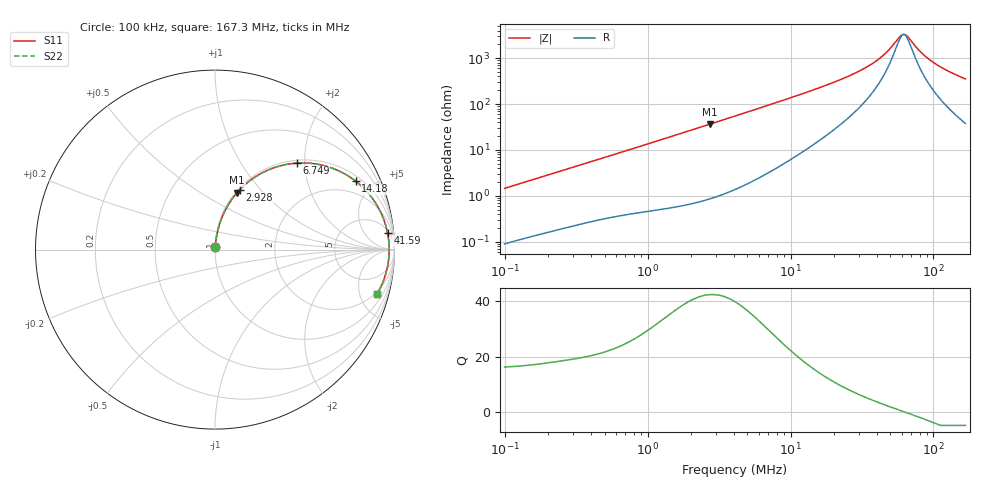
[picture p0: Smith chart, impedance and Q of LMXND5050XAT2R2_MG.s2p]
! LMXND5050XAT2R2_MG  S-PARAMETER MODEL  ( General Type )
! Model Generated by TAIYO YUDEN Corporation (https://www.yuden.co.jp/en/)
! Version 1.0
! TAIYO YUDEN Control No. 191023NI43SB-FBB
! Copyright(c) 2019 TAIYO YUDEN CO.,LTD. All Rights Reserved.
! Product Description (link to TY-COMPAS)
! https://ds.yuden.co.jp/TYCOMPAS/or/detail?pn=LMXND5050XAT2R2NMG&u=M
! Products Name : Inductors
! Characteristics :
!  Inductance : 2.2 uH , SRF(min) : 46 MHz , DC Resistance(max) : 0.0299 Ohm
!  Rated Current : Saturation :4200 mA , Temp Rise : 3500 mA (40 degC)
!  Case Size : 4.9 x 4.9 / 0.193 x 0.193 [mm/inch] , Thickness : 3.1 / 0.122 [mm/inch]
!  (Conditions: Temperature = 25 degC , DC Bias Current/Voltage = 0A / 0V)
! External Node Assignments :
!  1  o---GGG---o  2
! GND o---------o GND
! Frequency Range : 0.1MHz  -  167.251077MHz  [ 402 STEP ]
# MHz S RI R 50
! Freq[MHz].  S11 Real  S11 Imag  S21 Real  S21 Imag  S12 Real  S12 Imag  S22 Real  S22 Imag
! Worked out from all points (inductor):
!   401 points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, 100 kHz to 167.3 MHz, reference 50 ohm
!   read as one part in series: L = 2.29 uH near 103.8 kHz
!   highest Q = 42.5 at 2.719 MHz (marker M1), where L = 2.13 uH
!   self-resonance near 61.96 MHz
!   S11 on the Smith chart (normalised r, x): 100 kHz: 1.00, +0.03; 2.928 MHz: 1.02, +0.78; 6.749 MHz: 1.06, +1.82; 14.18 MHz: 1.25, +3.97; 41.59 MHz: 7, +18; 167.3 MHz: 1.75, -7.01
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0.1  0.00111 0.0145  0.9989 -0.0145  0.9989 -0.0145  0.00111 0.0145
0.346668  0.00474 0.0478  0.9953 -0.0478  0.9953 -0.0478  0.00474 0.0478
1.20179  0.03 0.1558  0.97 -0.1558  0.97 -0.1558  0.03 0.1558
2.718937  0.1225 0.3163  0.8775 -0.3163  0.8775 -0.3163  0.1225 0.3163
2.928417  0.1388 0.3342  0.8612 -0.3342  0.8612 -0.3342  0.1388 0.3342
4.166227  0.2431 0.4165  0.7569 -0.4165  0.7569 -0.4165  0.2431 0.4165
6.749349  0.4546 0.4818  0.5454 -0.4818  0.5454 -0.4818  0.4546 0.4818
9.602225  0.6267 0.4624  0.3733 -0.4624  0.3733 -0.4624  0.6267 0.4624
14.17747  0.7841 0.3811  0.2159 -0.3811  0.2159 -0.3811  0.7841 0.3811
19.43533  0.8707 0.2939  0.1293 -0.2939  0.1293 -0.2939  0.8707 0.2939
27.14211  0.9267 0.2008  0.0733 -0.2008  0.0733 -0.2008  0.9267 0.2008
34.54642  0.9504 0.138  0.0496 -0.138  0.0496 -0.138  0.9504 0.138
41.58984  0.9616 0.0925  0.0384 -0.0925  0.0384 -0.0925  0.9616 0.0925
49.14881  0.9676 0.0531  0.0324 -0.0531  0.0324 -0.0531  0.9676 0.0531
59.16942  0.9704 0.0105  0.0296 -0.0105  0.0296 -0.0105  0.9704 0.0105
61.40647  0.9705 0.00204  0.0295 -0.00204  0.0295 -0.00204  0.9705 0.00204
63.7281  0.9705 -0.00642  0.0295 0.00642  0.0295 0.00642  0.9705 -0.00642
67.37616  0.9702 -0.0191  0.0298 0.0191  0.0298 0.0191  0.9702 -0.0191
81.113  0.9666 -0.0619  0.0334 0.0619  0.0334 0.0619  0.9666 -0.0619
95.85533  0.9598 -0.1016  0.0402 0.1016  0.0402 0.1016  0.9598 -0.1016
124.2894  0.941 -0.1667  0.059 0.1667  0.059 0.1667  0.941 -0.1667
167.2511  0.9029 -0.2471  0.0971 0.2471  0.0971 0.2471  0.9029 -0.2471
